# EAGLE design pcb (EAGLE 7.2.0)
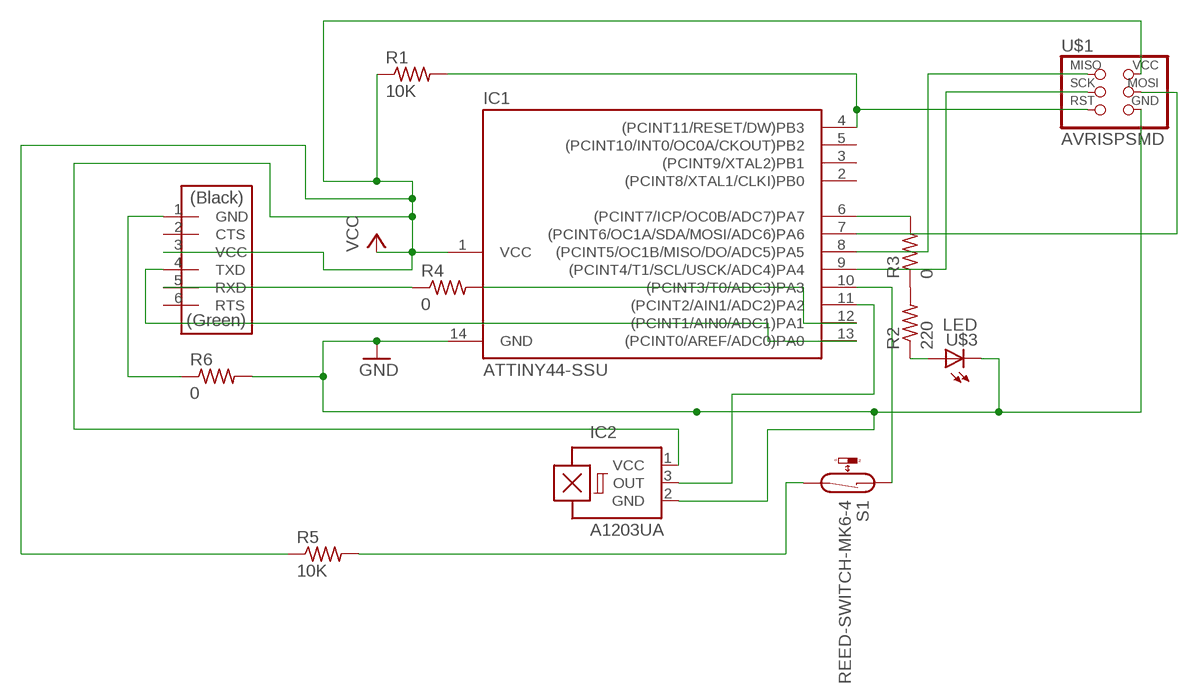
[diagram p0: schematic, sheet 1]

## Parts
IC1  ATTINY44-SSU  [SOIC14]
IC2  A1203UA  [SIP3-UA]
R1  10K  RES-US1206  [R1206]
R2  220  RES-US1206FAB  [R1206FAB]
R3  0  RES-US1206FAB  [R1206FAB]
R4  0  RES-US1206  [R1206]
R5  10K  RES-US1206  [R1206]
R6  0  RES-US1206FAB  [R1206FAB]
S1  REED-SWITCH-MK6-4  [MK6-4]
U$1  AVRISPSMD  [2X03SMD]
U$2  FTDI-SMD-HEADER  [1X06SMD]
U$3  LED  [LED1206]

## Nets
GND: IC1.14(GND) IC2.2(GND) R6.2 U$1.6(GND) U$3.2(C)
N$1: IC1.8((PCINT5/OC1B/MISO/DO/ADC5)PA5) U$1.1(MISO)
N$2: IC1.9((PCINT4/T1/SCL/USCK/ADC4)PA4) U$1.3(SCK)
N$3: IC1.4((PCINT11/RESET/DW)PB3) R1.2 U$1.5(RST)
N$4: R2.1 U$3.1(A)
N$5: IC1.6((PCINT7/ICP/OC0B/ADC7)PA7) R3.2
N$6: IC1.7((PCINT6/OC1A/SDA/MOSI/ADC6)PA6) U$1.4(MOSI)
N$7: R2.2 R3.1
N$8: IC1.12((PCINT1/AIN0/ADC1)PA1) R4.2
N$9: IC1.13((PCINT0/AREF/ADC0)PA0) U$2.4(TXD)
N$10: R4.1 U$2.5(RXD)
N$11: R5.2 S1.2
N$12: IC1.10((PCINT3/T0/ADC3)PA3) S1.1
N$13: IC1.11((PCINT2/AIN1/ADC2)PA2) IC2.3(OUT)
N$14: R6.1 U$2.1(GND)
VCC: IC1.1(VCC) IC2.1(VCC) R1.1 R5.1 U$1.2(VCC) U$2.3(VCC)
Unconnected: IC1.2((PCINT8/XTAL1/CLKI)PB0) IC1.3((PCINT9/XTAL2)PB1) IC1.5((PCINT10/INT0/OC0A/CKOUT)PB2) U$2.2(CTS) U$2.6(RTS)

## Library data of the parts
IC1 = fab:ATTINY44
IC2 = allegro:A12*?: Hall-effect bipolar switch Source: http://www.allegromicro.com/en/Products/Part_Numbers/1202/1202.pdf; OC_FARNELL: 1521672; OC_NEWARK: unknown
R1-R6 = fab:RES-US: Resistor (US Symbol)
S1 = switch-reed:REED-SWITCH-: Reed Sensor; OC_FARNELL: unknown
U$1 = fab:AVRISP
U$2 = fab:FTDI-SMD-HEADER
U$3 = fab:LED: LED

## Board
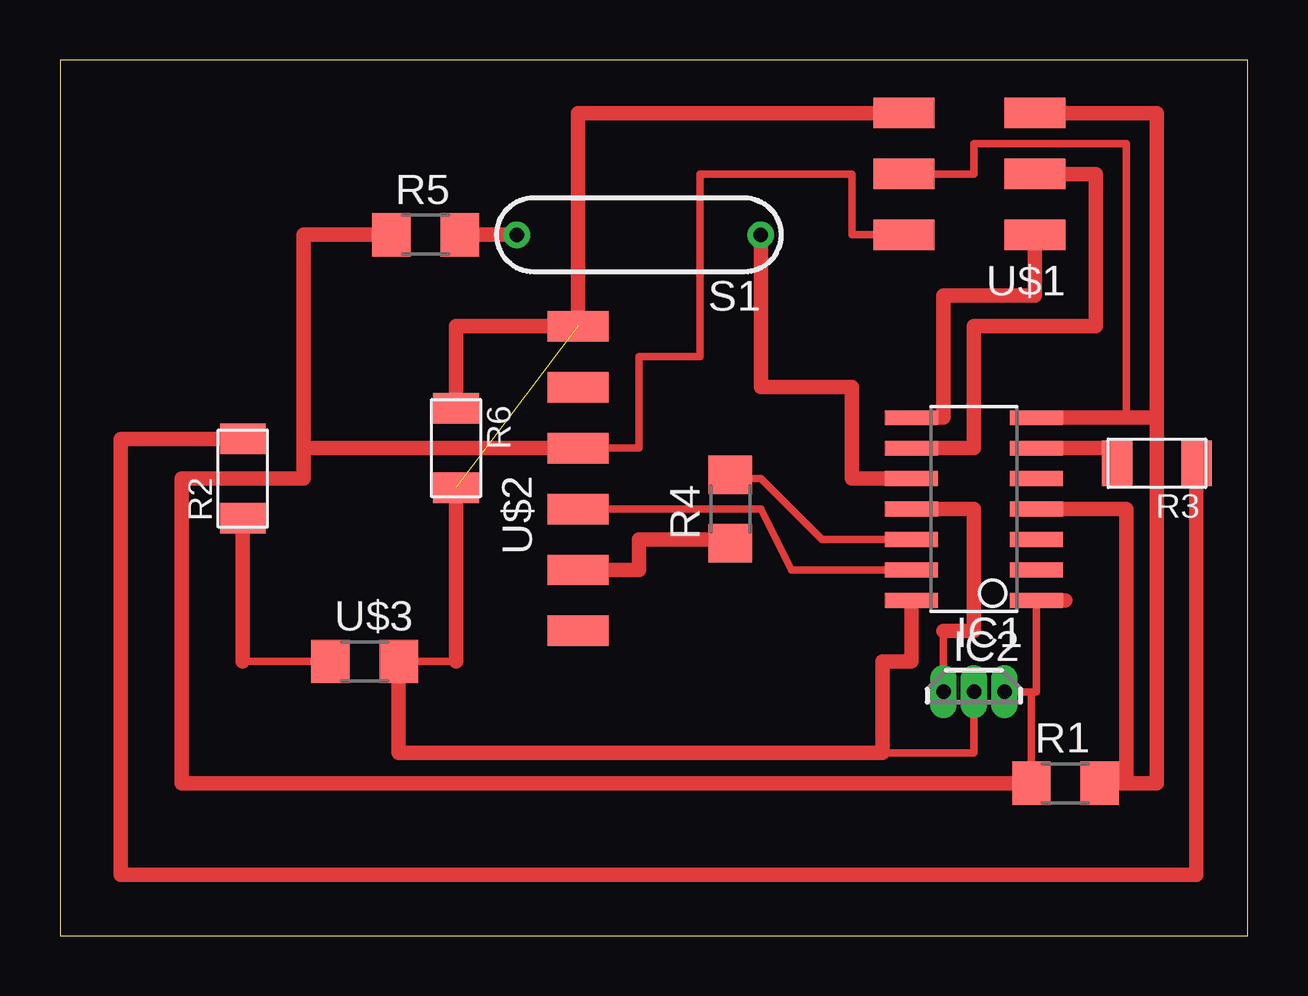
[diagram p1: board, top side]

Size 49.51 x 36.5 mm. Coordinates in mm from the lower left corner, seen from the top.
Outline: 0,0 49.51,0 49.51,36.5 0,36.5 0,0
Copper layers (1*16): Top 0.035mm / dielectric 1.5mm / Bottom 0.035mm
Design rules "default": minimum track width 10mil, minimum drill 24mil, track to track 8mil, track to pad 8mil, pad to pad 8mil, via to via 8mil, smd to smd 8mil, copper to edge 40mil, drill to drill 8mil, minimum pad ring 10mil, minimum via ring 8mil, stop-mask expansion 4mil, vias tented up to drill 0mil, thermal gap 10mil

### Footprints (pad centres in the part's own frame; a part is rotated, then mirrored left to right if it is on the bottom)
SOIC14 = smd 0.61 x 2.21: 1 -3.81,-2.603; 2 -2.54,-2.603; 3 -1.27,-2.603; 4 0,-2.603; 5 1.27,-2.603; 6 2.54,-2.603; 7 3.81,-2.603; 8 3.81,2.603; 9 2.54,2.603; 10 1.27,2.603; 11 0,2.603; 12 -1.27,2.603; 13 -2.54,2.603; 14 -3.81,2.603
SIP3-UA = drill 0.6 pad 0.7 long: 1 -1.27,0; 2 0,0; 3 1.27,0
R1206 = smd 1.6 x 1.803: 1 -1.422,0; 2 1.422,0
R1206FAB = smd 1.27 x 1.905: 1 -1.651,0; 2 1.651,0
MK6-4 = drill 0.6 pad 1.016: 1 -5.08,0; 2 5.08,0
2X03SMD = smd 2.54 x 1.27: 1 -2.54,2.54; 2 2.92,2.54; 3 -2.54,0; 4 2.92,0; 5 -2.54,-2.54; 6 2.92,-2.54
1X06SMD = smd 2.54 x 1.27: 1 0,6.35; 2 0,3.81; 3 0,1.27; 4 0,-1.27; 5 0,-3.81; 6 0,-6.35
LED1206 = smd 1.6 x 1.803: 1 -1.422,0; 2 1.422,0

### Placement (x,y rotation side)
IC1  38.1,17.78 90 top
IC2  38.1,10.16 180 top
R1  41.91,6.35 0 top
R2  7.62,19.05 90 top
R3  45.72,19.68 180 top
R4  27.94,17.78 90 top
R5  15.24,29.21 0 top
R6  16.51,20.32 270 top
S1  24.13,29.21 180 top
U$1  38.1,31.75 180 top
U$2  21.59,19.05 0 top
U$3  12.7,11.43 0 top

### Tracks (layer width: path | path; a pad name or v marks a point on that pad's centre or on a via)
GND  (1 unrouted)
  Top 0.305: IC2.2 38.1,7.62 34.29,7.62 | U$3.2 16.51,11.43
  Top 0.61: IC1.14 35.5,11.43 34.29,11.43 34.29,7.62 14.12,7.62 U$3.2 | 16.51,11.43 R6.2 | U$1.6 21.59,34.29 21.59,25.4
N$1
  Top 0.61: IC1.8 36.83,21.59 36.83,26.67 40.64,26.67 U$1.1
N$2
  Top 0.61: IC1.9 38.1,20.32 38.1,25.4 43.18,25.4 43.18,31.75 U$1.3
N$3
  Top 0.61: IC1.4 44.45,17.78 44.45,6.35 R1.2 45.72,6.35 45.72,34.29 U$1.5
N$4
  Top 0.305: U$3.1 7.62,11.43
  Top 0.61: 7.62,11.43 R2.1
N$5
  Top 0.61: IC1.6 44.07,20.32 R3.2
N$6
  Top 0.305: 44.45,21.59 44.45,33.02 38.1,33.02 38.1,31.75 U$1.4
  Top 0.61: 44.45,21.59 IC1.7 45.72,21.59 45.72,33.02
N$7
  Top 0.61: R2.2 2.54,20.7 2.54,2.54 47.37,2.54 R3.1
N$8
  Top 0.305: 28.09,19.05 29.21,19.05 31.75,16.51 IC1.12
  Top 0.61: R4.2 28.09,19.05
N$9
  Top 0.305: U$2.4 29.21,17.78 30.48,15.24 IC1.13
N$10
  Top 0.61: U$2.5 24.13,15.24 24.13,16.51 27.94,16.51 R4.1
N$11
  Top 0.61: S1.2 R5.2
N$12
  Top 0.61: S1.1 29.21,22.86 33.02,22.86 33.02,19.05 IC1.10
N$13
  Top 0.305: IC2.3 36.83,12.7
  Top 0.61: 36.83,12.7 38.1,12.7 38.1,17.78 IC1.11
N$14
  Top 0.61: R6.1 16.51,25.4 U$2.1
VCC
  Top 0.305: IC2.1 40.49,10.16 | IC1.1 40.7,10.16 40.49,10.16 | 40.49,10.16 R1.1 | U$1.2 33.02,29.21 33.02,31.75 26.67,31.75 26.67,24.13 24.13,24.13 24.13,20.32 U$2.3
  Top 0.61: IC1.1 41.91,13.97 | 10.16,20.32 10.16,29.21 R5.1 | 10.16,20.32 10.16,19.05 5.08,19.05 5.08,6.35 R1.1 | U$2.3 10.16,20.32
